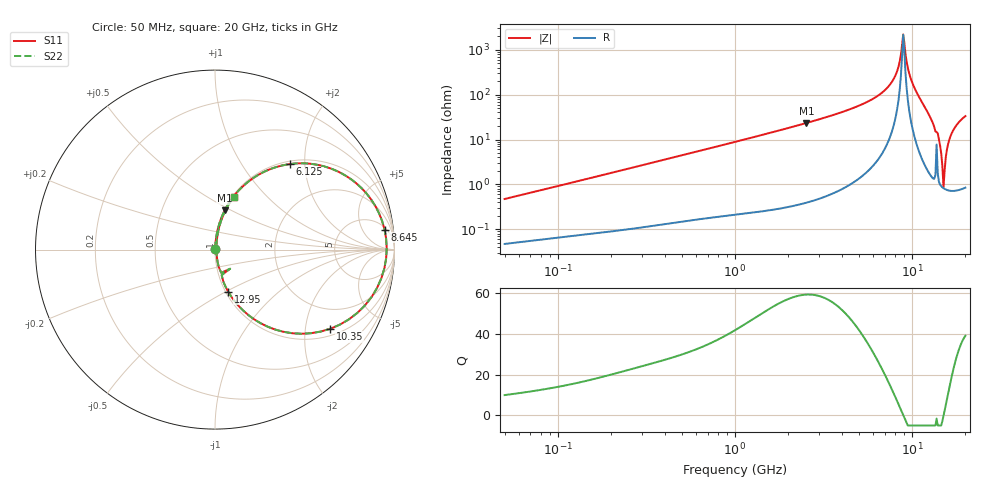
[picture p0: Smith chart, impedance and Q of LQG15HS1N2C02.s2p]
!Murata Part Number: LQG15HS1N2C02
!These Parameters are Measured in Series Mode Connection
!  o--[Z]--o
!Port1  Port2
!  o-------o
!Freq. Start=50[MHz] Stop=20[GHz], 401[Steps]
# Hz S RI R 50
!Freq.(Hz) S11(Real) S11(Imag) S21(Real) S21(Imag) S12(Real) S12(Imag) S22(Real) S22(Imag)
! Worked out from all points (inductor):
!   401 points, 50 MHz to 20 GHz, reference 50 ohm
!   read as one part in series: L = 1.49 nH near 51.52 MHz
!   highest Q = 59.4 at 2.531 GHz (marker M1), where L = 1.47 nH
!   self-resonance near 8.907 GHz
!   S11 on the Smith chart (normalised r, x): 50 MHz: 1.00, +0.01; 6.125 GHz: 1.06, +1.68; 8.645 GHz: 6, +14; 10.35 GHz: 1.22, -2.74; 12.95 GHz: 1.03, -0.51; 20 GHz: 1.02, +0.66
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5e7  0.000496 0.00471  0.9995 -0.00471  0.9995 -0.00471  0.000496 0.00471
1.364002e8  0.000908 0.0124  0.9991 -0.0124  0.9991 -0.0124  0.000908 0.0124
3.721004e8  0.00235 0.033  0.9977 -0.033  0.9977 -0.033  0.00235 0.033
1e9  0.0098 0.0873  0.9902 -0.0873  0.9902 -0.0873  0.0098 0.0873
2.531158e9  0.0548 0.2194  0.9452 -0.2194  0.9452 -0.2194  0.0548 0.2194
2.728004e9  0.0639 0.2363  0.9361 -0.2363  0.9361 -0.2363  0.0639 0.2363
4.472136e9  0.1885 0.3807  0.8115 -0.3807  0.8115 -0.3807  0.1885 0.3807
6.125241e9  0.4166 0.4765  0.5834 -0.4765  0.5834 -0.4765  0.4166 0.4765
7.442007e9  0.7075 0.4236  0.2925 -0.4236  0.2925 -0.4236  0.7075 0.4236
8.141811e9  0.8697 0.2796  0.1303 -0.2796  0.1303 -0.2796  0.8697 0.2796
8.644534e9  0.9448 0.1111  0.0552 -0.1111  0.0552 -0.1111  0.9448 0.1111
9.041845e9  0.9536 -0.0479  0.0464 0.0479  0.0464 0.0479  0.9536 -0.0479
9.600142e9  0.8726 -0.2639  0.1274 0.2639  0.1274 0.2639  0.8726 -0.2639
1.034674e10  0.6423 -0.441  0.3577 0.441  0.3577 0.441  0.6423 -0.441
1.295331e10  0.0735 -0.2344  0.9265 0.2344  0.9265 0.2344  0.0735 -0.2344
1.417136e10  0.0212 -0.098  0.9788 0.098  0.9788 0.098  0.0212 -0.098
1.460232e10  0.0113 -0.0473  0.9887 0.0473  0.9887 0.0473  0.0113 -0.0473
1.504638e10  0.00817 -0.00239  0.9918 0.00239  0.9918 0.00239  0.00817 -0.00239
1.550395e10  0.00918 0.0391  0.9908 -0.0391  0.9908 -0.0391  0.00918 0.0391
1.597544e10  0.0134 0.0777  0.9866 -0.0777  0.9866 -0.0777  0.0134 0.0777
1.670968e10  0.0246 0.1307  0.9754 -0.1307  0.9754 -0.1307  0.0246 0.1307
2e10  0.1055 0.2947  0.8945 -0.2947  0.8945 -0.2947  0.1055 0.2947
